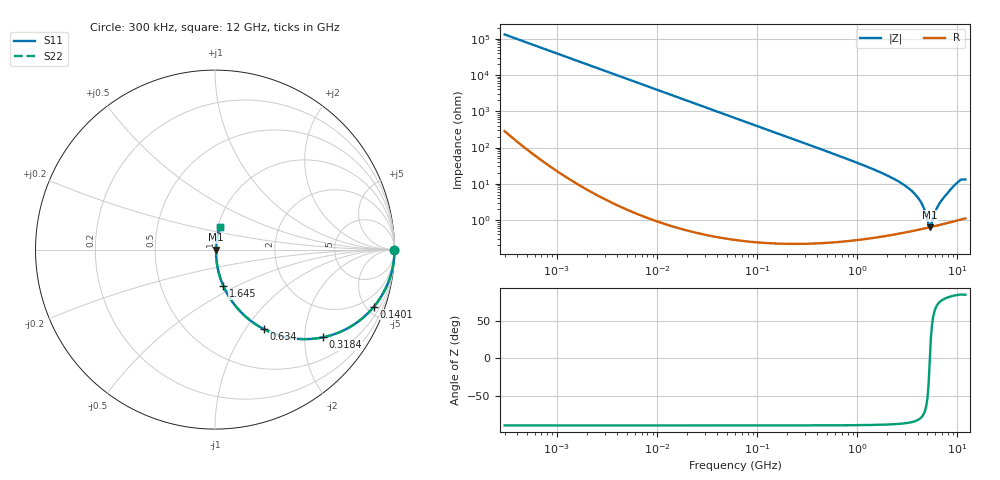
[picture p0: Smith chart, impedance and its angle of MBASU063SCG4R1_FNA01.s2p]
! MBASU063SCG4R1_FNA01  S-PARAMETER MODEL  ( General Type )
! Model Generated by TAIYO YUDEN Corporation (http://www.ty-top.com)
! Version 1.0
! TAIYO YUDEN Control No. 130801
! Copyright(c) 2013 TAIYO YUDEN CO.,LTD. All Rights Reserved.
! Product Description (link to TY-COMPAS)
! https://ds.yuden.co.jp/TYCOMPAS/or/detail?pn=MBASU063SCG4R1CFNA01&u=M
! Products Name : Multilayer Ceramic Capacitors
! Characteristics :
!  Capacitance : 4.1 pF , Rated Voltage : 50V , TCC : CG / C0G
!  Case Size : 0.6 x 0.3 / 0.024 x 0.012 [mm/inch] , Thickness : 0.3 / 0.012 [mm/inch]
!  (Conditions: Temperature = 25 degC , DC Bias Current/Voltage = 0A / 0V)
! External Node Assignments :
!  1  o---| |---o  2
! GND o---------o GND
! Frequency Range : 0.3MHz  -  12000MHz  [ 401 STEP ]
# MHz S RI R 50
! Freq[MHz].  S11 Real  S11 Imag  S21 Real  S21 Imag  S12 Real  S12 Imag  S22 Real  S22 Imag
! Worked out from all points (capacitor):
!   401 points, 300 kHz to 12 GHz, reference 50 ohm
!   read as one part in series: C = 4.06 pF near 316.3 kHz
!   lowest |Z| = 633 mohm at 5.279 GHz (marker M1)
!   series resonance near 5.297 GHz, so ESL is about 220 pH
!   S11 on the Smith chart (normalised r, x): 300 kHz: open; 140.1 MHz: 1.00, -5.59; 318.4 MHz: 1.00, -2.45; 634 MHz: 1.00, -1.22; 1.645 GHz: 1.01, -0.43; 12 GHz: 1.02, +0.26
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0.3  1 -0.000766  2.24e-06 0.000766  2.24e-06 0.000766  1 -0.000766
1.769972  1 -0.00452  2.21e-05 0.00452  2.21e-05 0.00452  1 -0.00452
10.44266  0.9993 -0.0266  0.000717 0.0266  0.000717 0.0266  0.9993 -0.0266
60  0.977 -0.1497  0.023 0.1497  0.023 0.1497  0.977 -0.1497
140.0606  0.8863 -0.3171  0.1137 0.3171  0.1137 0.3171  0.8863 -0.3171
208.3979  0.7785 -0.4147  0.2215 0.4147  0.2215 0.4147  0.7785 -0.4147
318.4019  0.6001 -0.489  0.3999 0.489  0.3999 0.489  0.6001 -0.489
353.9943  0.548 -0.4967  0.452 0.4967  0.452 0.4967  0.548 -0.4967
634.0297  0.2713 -0.4426  0.7287 0.4426  0.7287 0.4426  0.2713 -0.4426
994.7115  0.1279 -0.3303  0.8721 0.3303  0.8721 0.3303  0.1279 -0.3303
1645.489  0.0472 -0.2042  0.9528 0.2042  0.9528 0.2042  0.0472 -0.2042
2088.533  0.028 -0.1534  0.972 0.1534  0.972 0.1534  0.028 -0.1534
3026.31  0.012 -0.0858  0.988 0.0858  0.988 0.0858  0.012 -0.0858
3841.137  0.00749 -0.0478  0.9925 0.0478  0.9925 0.0478  0.00749 -0.0478
4502.883  0.00627 -0.0239  0.9937 0.0239  0.9937 0.0239  0.00627 -0.0239
5006.236  0.00614 -0.00836  0.9939 0.00836  0.9939 0.00836  0.00614 -0.00836
5278.635  0.00628 -0.000449  0.9937 0.000449  0.9937 0.000449  0.00628 -0.000449
5565.855  0.00653 0.00636  0.9935 -0.00636  0.9935 -0.00636  0.00653 0.00636
6354.153  0.00757 0.0222  0.9924 -0.0222  0.9924 -0.0222  0.00757 0.0222
7448.838  0.00976 0.0434  0.9902 -0.0434  0.9902 -0.0434  0.00976 0.0434
10236.47  0.0223 0.1103  0.9777 -0.1103  0.9777 -0.1103  0.0223 0.1103
12000  0.0273 0.126  0.9727 -0.126  0.9727 -0.126  0.0273 0.126
